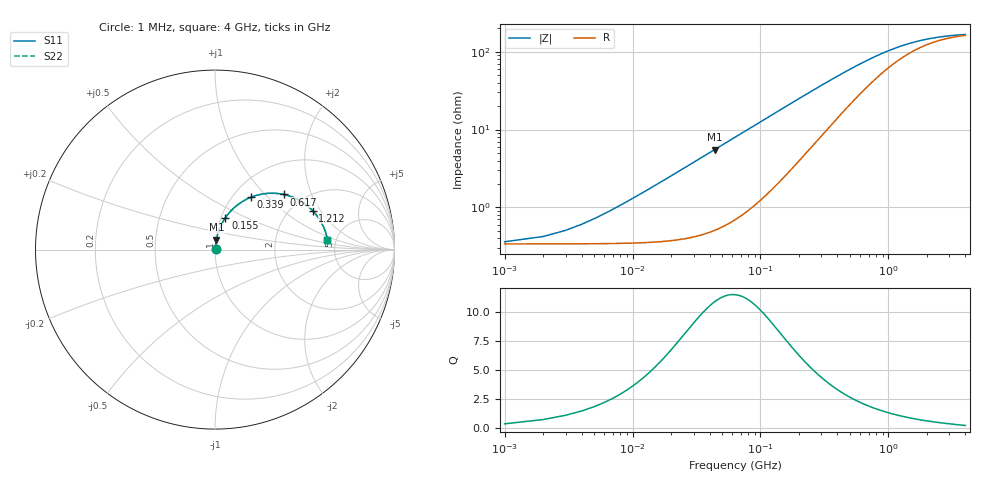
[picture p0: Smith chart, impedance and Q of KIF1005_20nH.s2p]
!version-2
!date-12.2020
!Series
# MHz S RI R 50
!Freq ReS11 ImS11 ReS21 ImS21 ReS12 ImS12 ReS22 ImS22
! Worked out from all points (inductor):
!   4000 points, 1 MHz to 4 GHz, reference 50 ohm
!   read as one part in series: L = 20 nH near 21 MHz
!   highest Q = 10.9 at 44 MHz (marker M1), where L = 20 nH
!   S11 on the Smith chart (normalised r, x): 1 MHz: 1.01, +0.00; 155 MHz: 1.05, +0.39; 339 MHz: 1.21, +0.81; 617 MHz: 1.60, +1.30; 1.212 GHz: 2.57, +1.70; 4 GHz: 4.25, +0.75
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1  0.00338 0.00125  0.9966 -0.00125  0.9966 -0.00125  0.00338 0.00125
10  0.00362 0.0125  0.9964 -0.0125  0.9964 -0.0125  0.00362 0.0125
23  0.00466 0.0286  0.9953 -0.0286  0.9953 -0.0286  0.00466 0.0286
27  0.00514 0.0336  0.9949 -0.0336  0.9949 -0.0336  0.00514 0.0336
35  0.00633 0.0435  0.9937 -0.0435  0.9937 -0.0435  0.00633 0.0435
44  0.00805 0.0545  0.992 -0.0545  0.992 -0.0545  0.00805 0.0545
63  0.0129 0.0775  0.9871 -0.0775  0.9871 -0.0775  0.0129 0.0775
88  0.0218 0.1068  0.9782 -0.1068  0.9782 -0.1068  0.0218 0.1068
118  0.036 0.1399  0.964 -0.1399  0.964 -0.1399  0.036 0.1399
155  0.0578 0.1772  0.9422 -0.1772  0.9422 -0.1772  0.0578 0.1772
235  0.1163 0.2416  0.8837 -0.2416  0.8837 -0.2416  0.1163 0.2416
339  0.2007 0.2918  0.7993 -0.2918  0.7993 -0.2918  0.2007 0.2918
462  0.2928 0.3132  0.7072 -0.3132  0.7072 -0.3132  0.2928 0.3132
617  0.3837 0.307  0.6163 -0.307  0.6163 -0.307  0.3837 0.307
668  0.4075 0.3008  0.5925 -0.3008  0.5925 -0.3008  0.4075 0.3008
909  0.4884 0.2633  0.5116 -0.2633  0.5116 -0.2633  0.4884 0.2633
1212  0.544 0.2172  0.456 -0.2172  0.456 -0.2172  0.544 0.2172
1334  0.5583 0.2013  0.4417 -0.2013  0.4417 -0.2013  0.5583 0.2013
2001  0.5995 0.1376  0.4005 -0.1376  0.4005 -0.1376  0.5995 0.1376
2667  0.6153 0.0988  0.3847 -0.0988  0.3847 -0.0988  0.6153 0.0988
3334  0.6227 0.0726  0.3773 -0.0726  0.3773 -0.0726  0.6227 0.0726
4000  0.6267 0.0534  0.3733 -0.0534  0.3733 -0.0534  0.6267 0.0534
